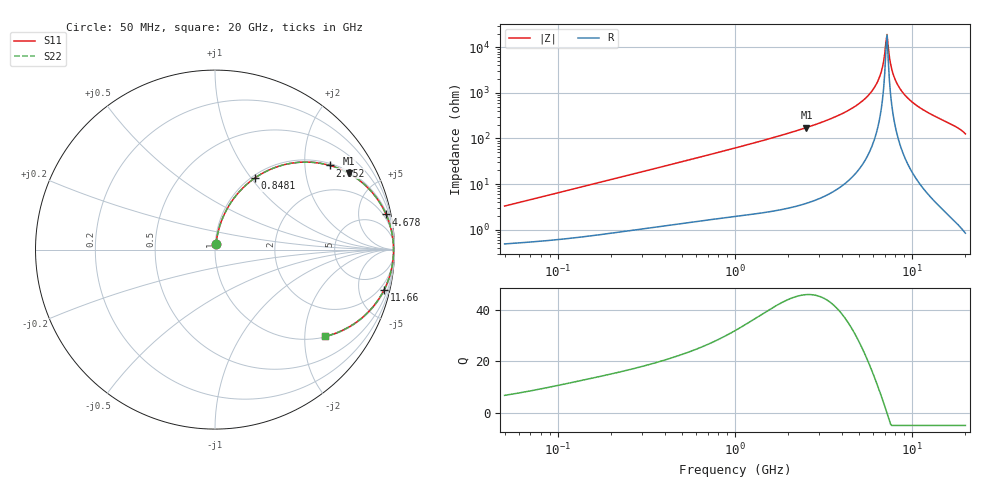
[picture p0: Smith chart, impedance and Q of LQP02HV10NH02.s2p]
!Murata Part Number: LQP02HV10NH02
!These Parameters are Measured in Series Mode Connection
!  o--[Z]--o
!Port1  Port2
!  o-------o
!Freq. Start=50[MHz] Stop=20[GHz], 401[Steps]
# Hz S RI R 50
!Freq.(Hz) S11(Real) S11(Imag) S21(Real) S21(Imag) S12(Real) S12(Imag) S22(Real) S22(Imag)
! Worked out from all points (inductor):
!   401 points, 50 MHz to 20 GHz, reference 50 ohm
!   read as one part in series: L = 10.3 nH near 51.52 MHz
!   highest Q = 45.8 at 2.531 GHz (marker M1), where L = 10.9 nH
!   self-resonance near 7.115 GHz
!   S11 on the Smith chart (normalised r, x): 50 MHz: 1.01, +0.07; 848.1 MHz: 1.04, +1.04; 2.052 GHz: 1.06, +2.68; 4.678 GHz: 1.31, +9.65; 11.66 GHz: 1.15, -8.31; 20 GHz: 1.02, -2.52
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5e7  0.00589 0.0323  0.9941 -0.0323  0.9941 -0.0323  0.00589 0.0323
1.364002e8  0.0142 0.0847  0.9858 -0.0847  0.9858 -0.0847  0.0142 0.0847
3.721004e8  0.0603 0.214  0.9397 -0.214  0.9397 -0.214  0.0603 0.214
8.480927e8  0.222 0.3988  0.778 -0.3988  0.778 -0.3988  0.222 0.3988
1e9  0.282 0.4346  0.718 -0.4346  0.718 -0.4346  0.282 0.4346
2.05233e9  0.6399 0.4689  0.3601 -0.4689  0.3601 -0.4689  0.6399 0.4689
2.531158e9  0.7454 0.4249  0.2546 -0.4249  0.2546 -0.4249  0.7454 0.4249
2.728004e9  0.7797 0.4036  0.2203 -0.4036  0.2203 -0.4036  0.7797 0.4036
4.677679e9  0.9531 0.196  0.0469 -0.196  0.0469 -0.196  0.9531 0.196
5.515528e9  0.9788 0.1225  0.0212 -0.1225  0.0212 -0.1225  0.9788 0.1225
6.217679e9  0.9899 0.0679  0.0101 -0.0679  0.0101 -0.0679  0.9899 0.0679
6.701223e9  0.9936 0.0334  0.00637 -0.0334  0.00637 -0.0334  0.9936 0.0334
7.009217e9  0.9947 0.0127  0.0053 -0.0127  0.0053 -0.0127  0.9947 0.0127
7.114996e9  0.9949 0.00573  0.00514 -0.00573  0.00514 -0.00573  0.9949 0.00573
7.331367e9  0.9949 -0.00816  0.00511 0.00816  0.00511 0.00816  0.9949 -0.00816
7.442007e9  0.9948 -0.0151  0.00524 0.0151  0.00524 0.0151  0.9948 -0.0151
7.784049e9  0.9938 -0.036  0.00623 0.036  0.00623 0.036  0.9938 -0.036
8.516016e9  0.9891 -0.0779  0.0109 0.0779  0.0109 0.0779  0.9891 -0.0779
9.745021e9  0.975 -0.1411  0.025 0.1411  0.025 0.1411  0.975 -0.1411
1.166392e10  0.9415 -0.2255  0.0585 0.2255  0.0585 0.2255  0.9415 -0.2255
1.646126e10  0.8112 -0.3869  0.1888 0.3869  0.1888 0.3869  0.8112 -0.3869
2e10  0.6132 -0.4837  0.3868 0.4837  0.3868 0.4837  0.6132 -0.4837
